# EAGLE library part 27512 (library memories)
EPROM 64K x 8 bits
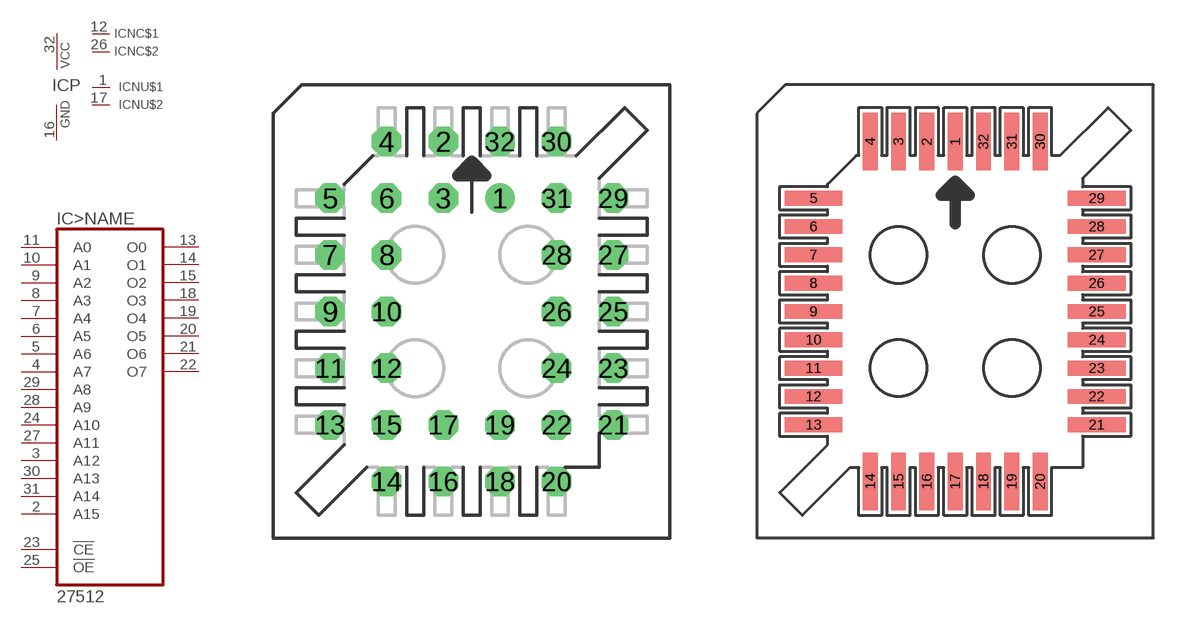
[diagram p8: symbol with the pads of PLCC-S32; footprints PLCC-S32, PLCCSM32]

Designator prefix IC; gates >NAME=27512 P=PWRN NC$1=NC NC$2=NC NU$1=NU NU$2=NU

## 27512S  [PLCC-S32]
1  NU$1:IC-NU  nc
2  >NAME:A15  in
3  >NAME:A12  in
4  >NAME:A7  in
5  >NAME:A6  in
6  >NAME:A5  in
7  >NAME:A4  in
8  >NAME:A3  in
9  >NAME:A2  in
10  >NAME:A1  in
11  >NAME:A0  in
12  NC$1:NC  nc
13  >NAME:O0  hiz
14  >NAME:O1  hiz
15  >NAME:O2  hiz
16  P:GND  pwr
17  NU$2:IC-NU  nc
18  >NAME:O3  hiz
19  >NAME:O4  hiz
20  >NAME:O5  hiz
21  >NAME:O6  hiz
22  >NAME:O7  hiz
23  >NAME:!CE  in
24  >NAME:A10  in
25  >NAME:!OE  in
26  NC$2:NC  nc
27  >NAME:A11  in
28  >NAME:A9  in
29  >NAME:A8  in
30  >NAME:A13  in
31  >NAME:A14  in
32  P:VCC  pwr

## 27512SMT  [PLCCSM32]
Pads as for PLCC-S32

## 27512  [PLCC32]
Pads as for PLCC-S32

## Footprint PLCC-S32 (pad centres in mm)
Plastic Leaded Chip Carrier Socket
drill 0.813: 1 1.27,5.08
drill 0.813 octagon: 2 -1.27,7.62; 3 -1.27,5.08; 4 -3.81,7.62; 5 -6.35,5.08; 6 -3.81,5.08; 7 -6.35,2.54; 8 -3.81,2.54; 9 -6.35,0; 10 -3.81,0; 11 -6.35,-2.54; 12 -3.81,-2.54; 13 -6.35,-5.08; 14 -3.81,-7.62; 15 -3.81,-5.08; 16 -1.27,-7.62; 17 -1.27,-5.08; 18 1.27,-7.62; 19 1.27,-5.08; 20 3.81,-7.62; 21 6.35,-5.08; 22 3.81,-5.08; 23 6.35,-2.54; 24 3.81,-2.54; 25 6.35,0; 26 3.81,0; 27 6.35,2.54; 28 3.81,2.54; 29 6.35,5.08; 30 3.81,7.62; 31 3.81,5.08; 32 1.27,7.62

## Footprint PLCCSM32 (pad centres in mm)
smd 0.66 x 2.591: 1 0,7.62; 2 -1.27,7.62; 3 -2.54,7.62; 4 -3.81,7.62; 14 -3.81,-7.62; 15 -2.54,-7.62; 16 -1.27,-7.62; 17 0,-7.62; 18 1.27,-7.62; 19 2.54,-7.62; 20 3.81,-7.62; 30 3.81,7.62; 31 2.54,7.62; 32 1.27,7.62
smd 2.591 x 0.66: 5 -6.35,5.08; 6 -6.35,3.81; 7 -6.35,2.54; 8 -6.35,1.27; 9 -6.35,0; 10 -6.35,-1.27; 11 -6.35,-2.54; 12 -6.35,-3.81; 13 -6.35,-5.08; 21 6.35,-5.08; 22 6.35,-3.81; 23 6.35,-2.54; 24 6.35,-1.27; 25 6.35,0; 26 6.35,1.27; 27 6.35,2.54; 28 6.35,3.81; 29 6.35,5.08

## Footprint PLCC32 (pad centres in mm)
PLASTIC LEADED CHIP CARRIER rectangle, package type L
smd 2.2 x 0.6: 1 -6.83,0; 2 -6.83,-1.27; 3 -6.83,-2.54; 4 -6.83,-3.81; 14 6.83,-3.81; 15 6.83,-2.54; 16 6.83,-1.27; 17 6.83,0; 18 6.83,1.27; 19 6.83,2.54; 20 6.83,3.81; 30 -6.83,3.81; 31 -6.83,2.54; 32 -6.83,1.27
smd 0.6 x 2.2: 5 -5.08,-5.56; 6 -3.81,-5.56; 7 -2.54,-5.56; 8 -1.27,-5.56; 9 0,-5.56; 10 1.27,-5.56; 11 2.54,-5.56; 12 3.81,-5.56; 13 5.08,-5.56; 21 5.08,5.56; 22 3.81,5.56; 23 2.54,5.56; 24 1.27,5.56; 25 0,5.56; 26 -1.27,5.56; 27 -2.54,5.56; 28 -3.81,5.56; 29 -5.08,5.56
